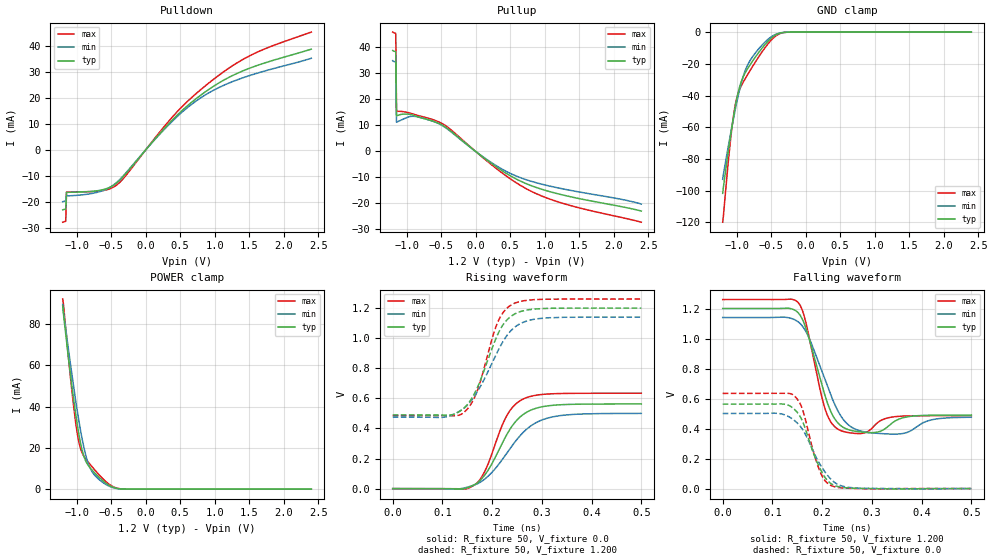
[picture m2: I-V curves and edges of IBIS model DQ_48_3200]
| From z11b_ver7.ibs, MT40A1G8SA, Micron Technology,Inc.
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| MODEL DQ_48_3200 (48 Ohm Data I/O with no ODT, 1600-3200Mbps)
[Model]   DQ_48_3200
Model_type   I/O
Vinl = 905.000mV
Vinh = 1015.000mV
Vmeas = 960.000mV
Vref = 1200.000mV
Cref = 0.0pF
Rref = 50.000Ohm
|   typ   min   max
|C_comp   0.810pF   0.760pF   0.860pF
C_comp_pullup   0.4050pF   0.3800pF   0.4300pF
C_comp_pulldown   0.4050pF   0.3800pF   0.4300pF
[Model Spec]
| Timing spec test load voltage corners
Vref   1.2000V   1.1400V   1.2600V
| Dynamic Overshoot Parameters from DDR4 Specification
|D_overshoot_ampl_h   0.40   NA   NA
|D_overshoot_ampl_l   0.40   NA   NA
|D_overshoot_area_h   0.0800n   NA   NA
|D_overshoot_area_l   0.0800n   NA   NA
[Voltage Range]   1.2000V   1.1400V   1.2600V
| Junction Temperature (Ambient temp is 35C typ, 95C min, 0C max)
[Temperature Range]   50.0   110.0   0.0
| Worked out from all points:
|   slope of the pulldown table from 0 to 0.18 V, typ, clamps not added: 32.4 ohm
|   slope of the pullup table from 0 to 0.18 V, typ, clamps not added: 49.2 ohm
|   GND clamp passes 1 mA (typ) near -0.39 V on its own axis
|   POWER clamp passes 1 mA (typ) near -0.48 V on its own axis
|   rising waveform, R_fixture 50, V_fixture 0.0: 20-80 % time 58.5ps typ, 73.9ps min, 46.5ps max; typ from 0 V to 0.563 V
|   falling waveform, R_fixture 50, V_fixture 1.200: 20-80 % time 36.2ps typ, 46ps min, 29.8ps max; typ from 1.2 V to 0.49 V
|   rising waveform, R_fixture 50, V_fixture 1.200: 20-80 % time 51.7ps typ, 64.2ps min, 42.1ps max; typ from 0.49 V to 1.2 V
|   falling waveform, R_fixture 50, V_fixture 0.0: 20-80 % time 38.7ps typ, 48.7ps min, 31.6ps max; typ from 0.563 V to 0 V
[Pulldown]
|   Voltage   I(typ)   I(min)   I(max)
-1.2V     -22.96mA   -19.84mA   -27.69mA
-1.156V   -22.64mA   -19.51mA   -27.34mA
-1.145V   -16.23mA   -17.61mA   -16.14mA
-698.2mV  -15.62mA   -16.21mA   -15.83mA
-545.5mV  -14.61mA   -14.73mA   -15.11mA
-414.5mV  -12.56mA   -12.33mA   -13.33mA
-305.5mV  -9.665mA   -9.372mA   -10.43mA
425.5mV   12.53mA    12.03mA    13.77mA
687.3mV   18.76mA    17.94mA    20.61mA
970.9mV   24.23mA    22.74mA    26.86mA
1.538V    31.71mA    28.84mA    36.56mA
2.4V      38.71mA    35.21mA    45.25mA
[GND_clamp]
|   Voltage   I(typ)   I(min)   I(max)
-1.2V     -101.7mA   -92.83mA   -119.9mA
-1.124V   -76.56mA   -73.18mA   -83.9mA
-1.08V    -63.49mA   -62.76mA   -65.41mA
-1.036V   -51.56mA   -52.83mA   -50.64mA
-992.7mV  -41.38mA   -43.58mA   -41.01mA
-927.3mV  -30.76mA   -31.6mA    -33.57mA
-872.7mV  -25.55mA   -24.13mA   -29.29mA
-818.2mV  -21.61mA   -19.01mA   -25.29mA
-621.8mV  -9.659mA   -7.8mA     -11.96mA
-436.4mV  -1.913mA   -1.476mA   -2.604mA
-229.1mV  -17.37uA   -20.1uA    -20.97uA
2.4V      0A         0A         0A
[Pullup]
|   Voltage   I(typ)   I(min)   I(max)
-1.2V     38.81mA    34.88mA    45.89mA
-1.156V   38.35mA    34.38mA    45.4mA
-1.145V   13.69mA    11.2mA     15.44mA
-905.5mV  13.92mA    13.51mA    14.37mA
-567.3mV  11.15mA    11.09mA    11.73mA
-370.9mV  8.067mA    7.853mA    8.629mA
0V        583.9nA    547.2nA    707.9nA
338.2mV   -6.633mA   -6.115mA   -7.357mA
600mV     -10.77mA   -9.589mA   -12.25mA
872.7mV   -13.81mA   -12mA      -16.18mA
1.375V    -17.43mA   -14.99mA   -20.83mA
2.4V      -22.93mA   -20.24mA   -27.22mA
[POWER_clamp]
|   Voltage   I(typ)   I(min)   I(max)
-1.2V     88.79mA    89.45mA    92.05mA
-1.189V   84.85mA    85.93mA    89.58mA
-1.135V   68.71mA    72.12mA    70.03mA
-1.047V   44.85mA    51mA       41.74mA
-1.004V   34.46mA    41.11mA    30.26mA
-960mV    25.41mA    31.92mA    21.99mA
-894.5mV  16.01mA    20.41mA    16.03mA
-807.3mV  10.49mA    10.53mA    12.15mA
-709.1mV  6.91mA     5.769mA    8.279mA
-534.5mV  1.991mA    1.551mA    2.56mA
-294.5mV  16.44uA    18.86uA    20.96uA
2.4V      0A         0A         0A
[Ramp]
|   typ   min   max
dV/dt_r   337.66m/58.45p   300.02m/73.86p   380.47m/46.54p
dV/dt_f   426.02m/36.24p   398.88m/45.99p   464.59m/29.78p
R_load = 50
[Rising Waveform]
R_fixture = 50
V_fixture = 0.0
|   Time   V(typ)   V(min)   V(max)
0s        2.71uV     9.036uV    1.603uV
137ps     -3.361mV   -115.1uV   -2.415mV
165ps     27.12mV    25.32mV    25.64mV
188ps     103.7mV    71.45mV    134.2mV
231ps     368.5mV    242.9mV    494mV
247ps     445.3mV    315.2mV    561.2mV
268ps     505.1mV    391.3mV    603.6mV
297ps     541.8mV    452.3mV    624.9mV
334ps     556.9mV    484.1mV    632mV
500ps     562.8mV    500mV      634.1mV
[Falling Waveform]
R_fixture   = 50
V_fixture   = 1.200
V_fixture_min = 1.140
V_fixture_max = 1.260
|   Time   V(typ)   V(min)   V(max)
0s        1.2V       1.14V      1.26V
152ps     1.171V     1.11V      1.239V
167ps     1.072V     1.049V     1.111V
206ps     617.2mV    722.5mV    529.3mV
236ps     423.6mV    492.2mV    388.4mV
262ps     384.5mV    403.5mV    368.8mV
304ps     373mV      369.8mV    415.6mV
342ps     440mV      362.8mV    477.4mV
422ps     488.9mV    459.3mV    485.6mV
500ps     490mV      475.2mV    485.7mV
[Rising Waveform]
R_fixture   = 50
V_fixture   = 1.200
V_fixture_min = 1.140
V_fixture_max = 1.260
|   Time   V(typ)   V(min)   V(max)
0s        490mV      475.8mV    485.7mV
104ps     488.2mV    475mV      485.6mV
145ps     540.2mV    539mV      511.4mV
170ps     669.6mV    643.2mV    649.6mV
211ps     1.024V     911.4mV    1.105V
226ps     1.107V     1V         1.187V
242ps     1.154V     1.064V     1.228V
269ps     1.186V     1.114V     1.252V
310ps     1.198V     1.135V     1.259V
500ps     1.2V       1.14V      1.26V
[Falling Waveform]
R_fixture = 50
V_fixture = 0.0
|   Time   V(typ)   V(min)   V(max)
0s        562.8mV    500.2mV    634.1mV
111ps     563.9mV    500.9mV    633.9mV
144ps     528.6mV    454.4mV    617.8mV
161ps     444.7mV    391.9mV    523mV
181ps     248mV      255.9mV    262mV
196ps     131.8mV    159.3mV    111.1mV
207ps     68.49mV    104.8mV    47.23mV
220ps     28.46mV    54.3mV     17.21mV
267ps     1.641mV    3.889mV    805uV
500ps     7.547uV    -89.51uV   7.457uV
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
